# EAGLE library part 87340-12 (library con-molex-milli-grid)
RECEPTACAL
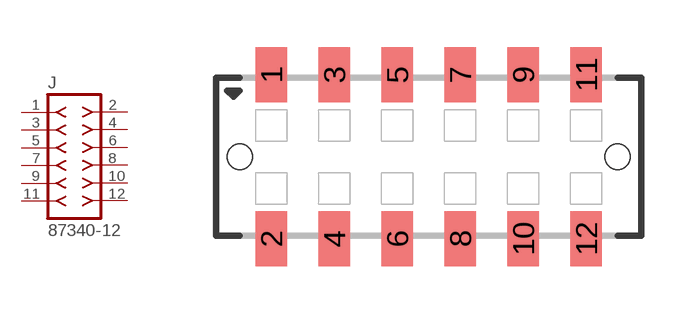
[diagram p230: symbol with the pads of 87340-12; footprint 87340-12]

Designator prefix J

## 87340-12  [87340-12]
1  1  pas
2  2  pas
3  3  pas
4  4  pas
5  5  pas
6  6  pas
7  7  pas
8  8  pas
9  9  pas
10  10  pas
11  11  pas
12  12  pas

## Footprint 87340-12 (pad centres in mm)
RECEPTACAL SMD Dual Row, Vertical, Low Profile
smd 1 x 1.75: 1 -5,2.6; 2 -5,-2.6; 3 -3,2.6; 4 -3,-2.6; 5 -1,2.6; 6 -1,-2.6; 7 1,2.6; 8 1,-2.6; 9 3,2.6; 10 3,-2.6; 11 5,2.6; 12 5,-2.6
hole 0.8 at -6,0
hole 0.8 at 6,0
